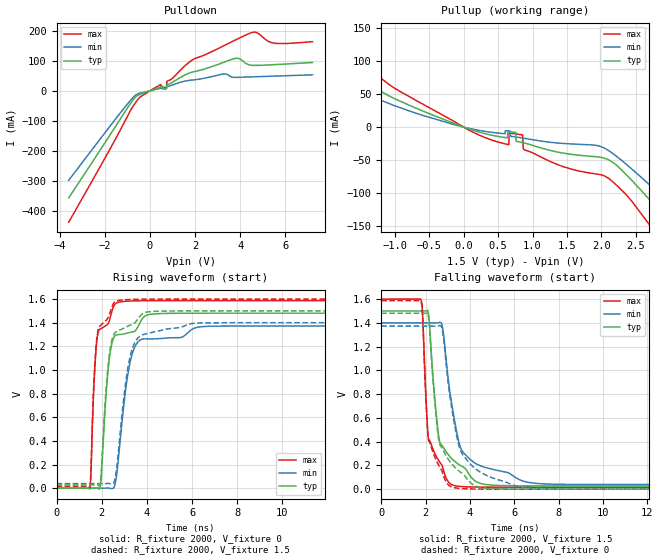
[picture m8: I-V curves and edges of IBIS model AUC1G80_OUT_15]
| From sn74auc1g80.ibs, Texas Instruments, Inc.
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[Model]   AUC1G80_OUT_15
Model_type  Output
Vref =   0
Rref =   2000
Cref =   15p
Vmeas =   0.75
| variable   typ   min   max
C_comp   6.96pF   1.51pF   19.46pF
| C_pullup   6.69pF   1.51pF   19.46pF
| C_pulldown   7.24pF   5.15pF   15.63pF
[Temperature Range]   40   100   -40
| Ambient temperature   25   85   -40
[Voltage range]   1.5   1.4   1.6
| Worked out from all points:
|   slope of the pulldown table from 0 to 0.225 V, typ, clamps not added: 36.4 ohm
|   slope of the pullup table from 0 to 0.225 V, typ, clamps not added: 29.5 ohm
|   rising waveform, R_fixture 2000, V_fixture 0: 20-80 % time 369ps typ, 544ps min, 246ps max; typ from 0 V to 1.48 V
|   falling waveform, R_fixture 2000, V_fixture 1.5: 20-80 % time 666ps typ, 789ps min, 436ps max; typ from 1.5 V to 0.027 V
|   rising waveform, R_fixture 2000, V_fixture 1.5: 20-80 % time 363ps typ, 535ps min, 240ps max; typ from 0.027 V to 1.5 V
|   falling waveform, R_fixture 2000, V_fixture 0: 20-80 % time 643ps typ, 839ps min, 414ps max; typ from 1.48 V to 0 V
[Pulldown]
| AUC1G80_OUT_15A
|   Voltage   I(typ)   I(min)   I(max)
-3.6V     -357.7mA   -298.8mA   -438.9mA
-845mV    -40mA      -30.15mA   -63.13mA
-410mV    -10.85mA   -7.015mA   -19.09mA
480mV     13.39mA    9.344mA    21.46mA
735mV     8.877mA    13.69mA    12.13mA
755mV     20.39mA    14.04mA    32.11mA
1.825V    61.58mA    35.93mA    100.8mA
3.275V    95.77mA    56.62mA    150.9mA
3.725V    107.6mA    45.07mA    167.8mA
4.505V    85.77mA    46.79mA    194.8mA
5.5V      87.65mA    49.31mA    159.6mA
7.2V      94.84mA    53.6mA     164.5mA
[Pullup]
| AUC1G80_OUT_15A
|   Voltage   I(typ)   I(min)   I(max)
-3.6V     254.3mA    195.3mA    304.9mA
-2.88V    188.1mA    148.5mA    234.4mA
-2.055V   116.2mA    88.7mA     153.6mA
85mV      -3.131mA   -2.055mA   -4.98mA
650mV     -6.785mA   -5.763mA   -26.6mA
660mV     -6.906mA   -5.859mA   -8.85mA
855mV     -23.44mA   -16.5mA    -11.77mA
885mV     -24.19mA   -17.02mA   -34.59mA
2.11V     -49.85mA   -35.9mA    -78.1mA
2.77V     -118mA     -94.08mA   -158.2mA
3.37V     -188.1mA   -152.5mA   -242.4mA
7.2V      -634.8mA   -537mA     -765.5mA
[Ramp]
| AUC1G80_OUT_15A
| variable   typ   min   max
dV/dt_r   0.89/3.69E-10   0.83/5.45E-10   0.96/2.46E-10
dV/dt_f   0.89/6.63E-10   0.82/7.86E-10   0.95/4.36E-10
R_load = 2000
[Rising Waveform]
| AUC1G80_OUT_15A
R_fixture =   2000
C_fixture =   0
L_fixture =   0
V_fixture =   0
V_fixture_min = 0
V_fixture_max = 0
|   Time   V(typ)   V(min)   V(max)
0s        7.268nV    27.24nV    884.6pV
1.47ns    -2.941uV   -2.939uV   -6.339mV
1.515ns   -1.765uV   -3.843uV   90.44mV
1.72ns    390.7uV    -4.611uV   1.098V
1.925ns   3.097mV    5.911uV    1.347V
2.315ns   1.056V     1.285mV    1.401V
2.69ns    1.299V     158.5mV    1.569V
3.215ns   1.317V     1.027V     1.583V
3.78ns    1.429V     1.26V      1.586V
21.42ns   1.481V     1.373V     1.587V
[Falling Waveform]
| AUC1G80_OUT_15A
R_fixture =   2000
C_fixture =   0
L_fixture =   0
V_fixture =   1.5
V_fixture_min = 1.4
V_fixture_max = 1.6
|   Time   V(typ)   V(min)   V(max)
0s        1.5V       1.4V       1.6V
1.785ns   1.5V       1.4V       1.599V
1.86ns    1.5V       1.4V       1.496V
2.13ns    1.474V     1.4V       425.6mV
2.61ns    422.9mV    1.403V     236mV
2.78ns    358.3mV    1.344V     179.4mV
3.235ns   247.6mV    656.7mV    34.05mV
4.01ns    112.7mV    251.5mV    18.92mV
6.645ns   27.7mV     56.91mV    16.5mV
21.42ns   27.21mV    38.78mV    16.41mV
[Rising Waveform]
| AUC1G80_OUT_15A
R_fixture =   2000
C_fixture =   0
L_fixture =   0
V_fixture =   1.5
V_fixture_min = 1.4
V_fixture_max = 1.6
|   Time   V(typ)   V(min)   V(max)
0s        27.17mV    38.77mV    16.4mV
1.47ns    27.17mV    38.77mV    10.26mV
1.515ns   27.17mV    38.77mV    109.1mV
1.72ns    27.55mV    38.77mV    1.123V
1.925ns   32.37mV    38.78mV    1.373V
2.305ns   1.074V     40.15mV    1.45V
2.665ns   1.327V     175.9mV    1.584V
3.21ns    1.376V     1.073V     1.596V
3.82ns    1.478V     1.298V     1.599V
21.42ns   1.5V       1.4V       1.6V
[Falling Waveform]
| AUC1G80_OUT_15A
R_fixture =   2000
C_fixture =   0
L_fixture =   0
V_fixture =   0
V_fixture_min = 0
V_fixture_max = 0
|   Time   V(typ)   V(min)   V(max)
0s        1.481V     1.373V     1.587V
1.785ns   1.481V     1.373V     1.586V
1.86ns    1.481V     1.373V     1.482V
2.125ns   1.459V     1.373V     418.1mV
2.59ns    420.9mV    1.375V     203.1mV
2.775ns   334.2mV    1.319V     136mV
3.175ns   214.4mV    689.1mV    19.08mV
3.95ns    68.13mV    226.5mV    2.635mV
6.24ns    689.4uV    18.93mV    125.2uV
21.42ns   34.59uV    9.811uV    14.69uV
